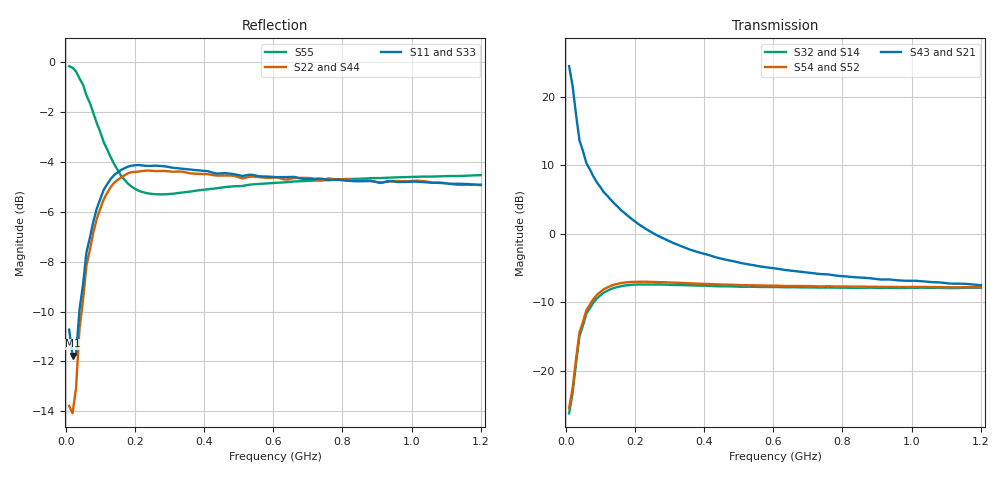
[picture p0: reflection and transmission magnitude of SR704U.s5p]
!  POLYFET RF DEVICES
!  S PARAMETERS FOR
!  SR704U (EACH SIDE)
!  VDS=28, IDQ=800MA
! S1A4+4Die, AR pkg, left side, Vds=28Vdc, Idq=800ma, Vgsth=2.63Vdc,
! Date: Mon Jul 27 15:55:45 1998
!AWR Design Environment (2053) Wed Feb 04 15:42:08 2004
!freq-unit  param-type  data-format  keyword  impedance-ohms
# MHz  S  MA  R  50
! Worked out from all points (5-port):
!   120 points, 10 MHz to 1.2 GHz, reference 50 ohm
!   strongest paths, dB at 10 MHz, 310 MHz, 610 MHz, 910 MHz, 1.2 GHz:
!     S43: 24.5, -1.3, -5.1, -6.7, -7.5
!     S21: 24.5, -1.3, -5.1, -6.7, -7.5
!     S54: -25.5, -7.2, -7.6, -7.8, -7.8
!     S52: -25.5, -7.2, -7.6, -7.8, -7.8
!     S32: -26.2, -7.5, -7.8, -7.9, -7.9
!     S14: -26.2, -7.5, -7.8, -7.9, -7.9
!   lowest |S11| = -11.8 dB at 20 MHz (marker M1), VSWR 1.70, Z = 49.8 - j26.6 ohm
!   |S11| at or under -10 dB: start of sweep to 39.59 MHz
